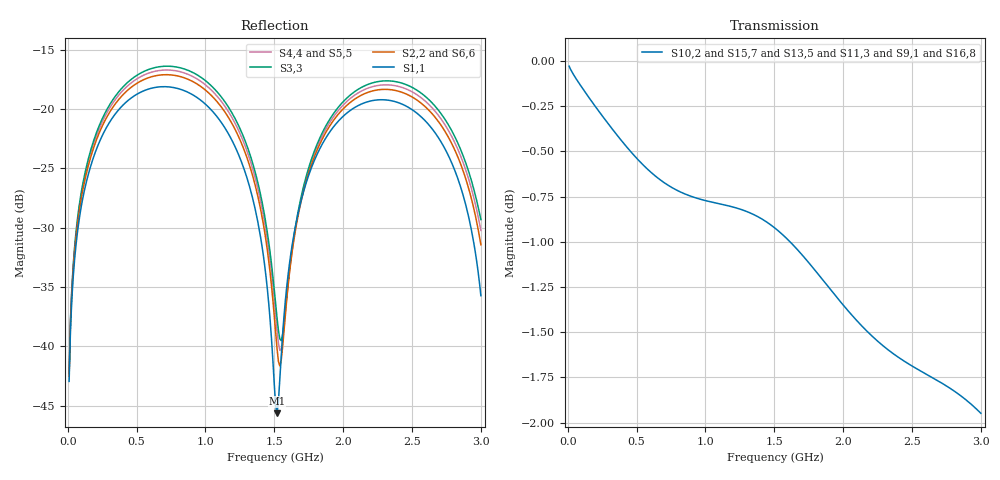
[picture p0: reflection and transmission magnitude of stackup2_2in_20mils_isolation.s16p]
! Touchstone file from project
# GHZ S RI R 50.000000
! Modal data exported
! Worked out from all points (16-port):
!   300 points, 10 MHz to 3 GHz, reference 50 ohm
!   strongest paths, dB at 10 MHz, 760 MHz, 1.51 GHz, 2.26 GHz, 3 GHz:
!     S10,2: 0.0, -0.7, -0.9, -1.6, -1.9
!     S15,7: 0.0, -0.7, -0.9, -1.6, -2.0
!     S13,5: 0.0, -0.7, -0.9, -1.6, -2.0
!     S11,3: 0.0, -0.7, -0.9, -1.6, -2.0
!     S9,1: 0.0, -0.7, -0.9, -1.5, -1.9
!     S16,8: 0.0, -0.7, -0.9, -1.5, -1.9
!   lowest |S11| = -45.6 dB at 1.52 GHz (marker M1), VSWR 1.01, Z = 50.5 - j0.0115 ohm
!   |S11| at or under -10 dB: start of sweep to end of sweep
